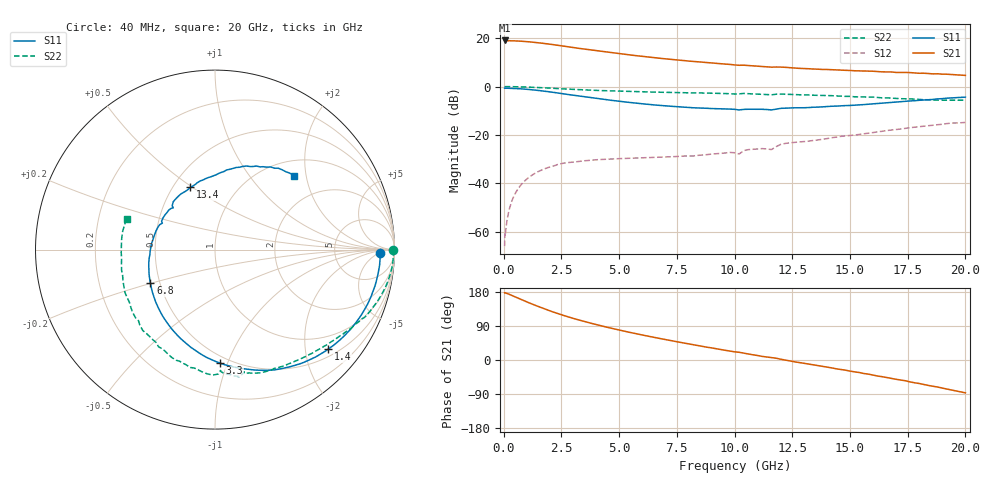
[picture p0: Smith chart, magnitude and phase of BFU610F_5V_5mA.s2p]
! Filename:  P:\Prog\Test\Noise\ATS_data\Testdata_Net\SplitFiles\BFU610_2W_A5_HighFreq_5V_5mA_D.s2p
! Date/Time: Wed 10/Aug/2011 16:58:18
! BFU610_2W_A5_HighFreq_5V_1mA_10mA_Bias3_R.s2p
! MDIF S-parameter v. bias file
! BFU610_2W_A5_HighFreq_5V_1mA_10mA
! Date/time Mon Aug 08 14:15:19 2011
! VAR V_out= 5.0000
! VAR I_out= 4.9950
! VAR V_in= 0.8775
! VAR I_in= 0.0380
! Device data file deembeded for feedlines and parallel
! Original file: \SplitFiles\BFU610_2W_A5_HighFreq_5V_5mA_R.s2p
! Feed-files: PR003V01_101208_Feed1.s2p, PR003V01_101208_Feed2.s2p
! Parallel-file: PR003V01_101208_Par.s2p
# MHz S MA R 50
!  Freq-MHz  S11-mag  S11-arg  S21-mag  S21-arg  S12-mag  S12-arg  S22-mag  S22-arg
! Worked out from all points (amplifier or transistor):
!   167 points, 40 MHz to 20 GHz, reference 50 ohm
!   highest |S21| = 19.0 dB at 40 MHz (marker M1)
!   |S21| within 3 dB of that: start of sweep to 3.068 GHz
!   unconditionally stable (mu >= 1): 5.558 GHz to 16.1 GHz; 16.34168 GHz to 16.40568 GHz
!   at 550 MHz: K = 0.06, MSG = 31.1 dB, |S12| = -43.4 dB
!   at 4.2 GHz: K = 0.73, MSG = 22.4 dB, |S12| = -30.2 dB
!   at 20 GHz: K = 0.74, MSG = 9.7 dB, |S12| = -14.8 dB
!   S11 on the Smith chart (normalised r, x): 40 MHz: 23, -5; 1.4 GHz: 0.66, -2.50; 3.3 GHz: 0.45, -0.94; 6.8 GHz: 0.44, -0.20; 13.4 GHz: 0.61, +0.49; 20 GHz: 1.32, +1.71
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40  0.9218 -1.1  8.941 177.4  0.000504 69.5  0.9923 -0.2
50  0.9162 -1.2  8.889 177.7  0.0008931 102.8  0.9929 -0.3
140  0.9214 -4.2  8.837 175.8  0.001662 84.8  0.9944 -1.5
380  0.9153 -11.6  8.791 169.6  0.004681 84.7  0.9926 -4.5
950  0.8808 -28.6  8.502 154.6  0.01168 74.7  0.977 -11.1
1400  0.8398 -41.4  8.104 143.5  0.01656 67.0  0.9575 -16.0
1850  0.7926 -53.5  7.651 133.0  0.02064 60.1  0.9349 -20.5
2250  0.7479 -63.7  7.212 124.3  0.02358 55.7  0.9143 -24.5
2800  0.6827 -76.5  6.619 113.7  0.02695 47.2  0.8823 -28.7
3300  0.6333 -87.4  6.105 104.9  0.02855 43.6  0.8586 -32.6
3400  0.6239 -89.5  6.018 103.2  0.02891 42.9  0.8548 -33.3
4100  0.5614 -103.8  5.428 92.0  0.03091 38.5  0.8286 -38.1
4900  0.5027 -118.8  4.84 80.5  0.03224 35.4  0.8046 -43.4
5800  0.45 -135.2  4.303 68.5  0.0334 33.6  0.7825 -49.3
6800  0.4057 -152.5  3.818 56.4  0.03466 33.4  0.7622 -55.7
8600  0.3573 177.9  3.191 36.2  0.03846 37.2  0.7357 -67.4
10200  0.3284 153.3  2.747 20.4  0.04029 41.9  0.7038 -76.6
12000  0.3538 131.1  2.52 2.1  0.06374 47.2  0.6988 -90.9
13400  0.3736 111.5  2.298 -12.6  0.07678 37.5  0.6611 -104.2
16800  0.4723 75.6  1.998 -48.6  0.1264 19.3  0.5772 -142.7
18800  0.5552 56.0  1.833 -71.4  0.1628 1.5  0.5227 -174.9
20000  0.6035 43.1  1.697 -86.7  0.1812 -12.0  0.5217 160.7
